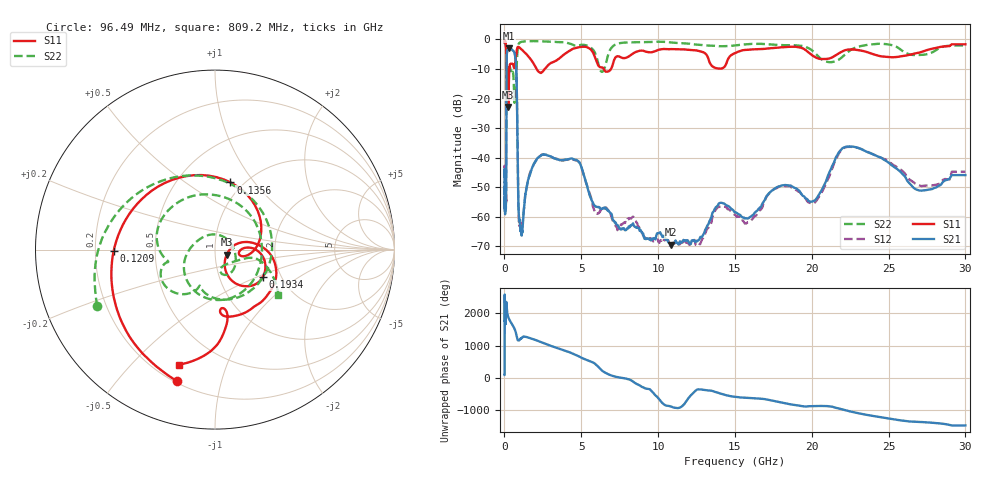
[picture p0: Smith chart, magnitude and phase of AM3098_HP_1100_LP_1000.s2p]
! Date/Time: Thu, Feb 28, 2019 8:44 AM
! Network Analyzer: Agilent Technologies E8364B Rev: A.07.50.67
! Sweep from 0.010 to 30.000 GHz, 1601 Points, Sweep Type: LOG
! Power Supply: 5.023 V, 0.002 A
# Hz S DB R 50
!freq MagS11 AngS11 MagS21 AngS21 MagS12 AngS12 MagS22 AngS22
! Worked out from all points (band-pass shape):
!   1601 points, 10 MHz to 30 GHz, reference 50 ohm
!   highest |S21| = -3.00 dB at 266.5 MHz (marker M1); lowest = -69.6 dB at 10.81 GHz (marker M2)
!   |S21| within 3 dB of the highest: 149.2 MHz to 706.3 MHz (557.2 MHz wide, 130 % of centre)
!   lowest |S11| = -22.9 dB at 248.4 MHz (marker M3), VSWR 1.15, Z = 56.9 - j3.33 ohm
!   |S11| at or under -10 dB: 140 MHz to 316.3 MHz (176.3 MHz wide, 77.3 % of centre); 2.093 GHz to 2.62 GHz (527.8 MHz wide, 22.4 % of centre); 6.476 GHz to 6.933 GHz (457.1 MHz wide, 6.82 % of centre)
!   |S22| runs from -21.5 to -0.5 dB; largest |S21 - S12| = 0.013
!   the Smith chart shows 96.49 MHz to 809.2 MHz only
!   S11 on the Smith chart (normalised r, x): 96.49 MHz: 0.21, -0.73; 120.9 MHz: 0.28, -0.01; 135.6 MHz: 0.87, +0.77; 193.4 MHz: 1.61, -0.55; 809.2 MHz: 0.30, -0.69
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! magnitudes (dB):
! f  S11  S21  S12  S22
! 10 MHz  -0.4  -46.5  -43.6  -0.6
! 38.04 MHz  -0.4  -56.7  -56.8  -0.8
! 96.49 MHz  -2.3  -55.1  -51.8  -2.8
! 109.9 MHz  -3.5  -51.7  -54.5  -4.1
! 120.9 MHz  -5.0  -36.3  -35.9  -6.5
! 135.6 MHz  -8.3  -13.9  -13.9  -10.1
! 144.7 MHz  -12.3  -7.4  -7.3  -11.4
! 193.4 MHz  -10.3  -3.6  -3.6  -9.3
! 248.4 MHz  -22.9  -3.0  -3.0  -11.4
! 266.5 MHz  -17.9  -3.0  -3.0  -11.2
! 550.5 MHz  -8.4  -3.8  -3.8  -11.1
! 655.8 MHz  -9.4  -4.5  -4.5  -21.5
! 809.2 MHz  -3.5  -18.9  -18.9  -7.2
! 917.1 MHz  -2.5  -57.7  -58.6  -1.5
! 1.082 GHz  -3.2  -65.1  -64.5  -0.8
! 2.084 GHz  -9.9  -40.7  -40.8  -0.6
! 4.734 GHz  -2.8  -41.0  -41.1  -2.1
! 7.926 GHz  -6.2  -64.5  -61.9  -1.0
! 10.81 GHz  -3.3  -69.6  -69.8  -1.0
! 20.1 GHz  -5.6  -54.7  -55.5  -4.1
! 22.56 GHz  -3.4  -36.3  -36.4  -3.5
! 30 GHz  -1.6  -45.9  -44.8  -2.1
